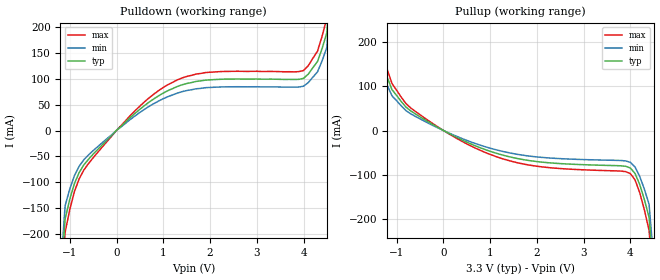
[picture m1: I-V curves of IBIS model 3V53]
[IBIS Ver]   2.1
[File name]   171601_3.ibs
[File Rev]   2.0
[Date]   8/4/03
[Source]   ICS MicroClock Applications Engineering 2
[Disclaimer] This information is for modeling purposes only, and is
(C) Copyright Integrated Circuit Systems, Inc. 1997-2003
   All rights reserved
ICS hereby grants the user of this IBIS model a non-exclusive,
nontransferable license to use this IBIS model under the following terms.
Before using this IBIS model, the user should read this license.
If the user does not accept these terms,  the IBIS model should be
returned to ICS within 30 days.
   The user is granted this license only to use the IBIS model and
is not granted rights to sell, load, rent, lease or license the IBIS
model in whole or in part, or in modified form to anyone other than
user. User may modify the IBIS model to suit its specific
applications but rights to derivative works and such modifications
shall belong to ICS.
   This IBIS model is provided on an "AS IS" basis and ICS makes
absolutely no warranty with respect to the information contained
herein. ICS DISCLAIMS AND CUSTOMER WAIVES ALL WARRANTIES, EXPRESS
OR IMPLIED, INCLUDING WARRANTIES OF MERCHANTABILITY OR FITNESS FOR
A PARTICULAR PURPOSE. The entire risk as to quality and performance
is with the Customer. ACCORDINGLY, IN NO EVENT SHALL THE COMPANY BE
LIABLE FOR ANY DAMAGES, WHETHER IN CONTRACT OR TORT,INCLUDING ANY
LOST PROFITS OR OTHER INCIDENTAL, CONSEQUENTIAL, EXEMPLARY, OR
PUNITIVE DAMAGES ARISING OUT OF THE USE OR APPLICATION OF THE IBIS
model provided in this package. Further, ICS reserves the right to
make changes without notice to any product herein to improve
reliability, function, or design. ICS does not convey any license
under patent rights or any other intellectual property rights,
including those of third parties.
   ICS is not obligated to provide maintenance or support
for the licensed IBIS model.
[Component]   MK1716-01
[Manufacturer] Integrated Circuit Systems Inc.
[Package]
|   typ   min   max
R_pkg   40m   35m   45m
L_pkg   1.65nH   1.35nH   1.95nH
C_pkg   0.24pF   0.14pF   0.34pF
[pin]   signal_name   model_name   R_pin   L_pin   C_pin
   4   REFOUT   3V53
  10   CLKA   3V53
  11   CLKA   3V53
  12   CLKA   3V53
  13   CLKA   3V53
  16   CLKB   3V53
  17   CLKB   3V53
  18   CLKB   3V53
  19   CLKB   3V53
| Models and submodels in the file (1): 3V53 (Output)
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|   MK1716-01 3.3V Clock Drive Model
| This model is suitable for all output pins on the
| MK1716-01
[Model]   3V53
Model_type   Output
Polarity   Non-Inverting
|   typ   min   max
C_comp   5pF   4pF   6pF
|   typ   min   max
[Voltage range]  3.3V   3.15V   3.45V
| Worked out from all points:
|   slope of the pulldown table from 0 to 0.495 V, typ, clamps not added: 12.3 ohm
|   slope of the pullup table from 0 to 0.495 V, typ, clamps not added: 18.9 ohm
[pulldown]
|Voltage   I (typ)   I (min)   I (max)
-3.3V     -3A        -3A        -3A
-1.1V     -170.4mA   -144.9mA   -196mA
-900mV    -102mA     -86.67mA   -117.3mA
-600mV    -55.36mA   -47.06mA   -63.66mA
500mV     41.05mA    34.89mA    47.2mA
1.3V      84.84mA    72.12mA    97.57mA
2V        97.7mA     83.04mA    112.4mA
4V        100.5mA    85.44mA    115.6mA
4.3V      133.1mA    113.2mA    153.1mA
4.4V      158.6mA    134.8mA    182.4mA
4.5V      188.8mA    160.5mA    217.1mA
6.6V      3A         3A         3A
[pullup]
|Voltage I (typ)   I (min)   I (max)
-3.3V     3A         3A         3A
-1.5V     200.2mA    170.1mA    230.2mA
-1.4V     182.5mA    155.1mA    209.8mA
-1.1V     92.5mA     78.62mA    106.4mA
-800mV    52.88mA    44.95mA    60.82mA
400mV     -21.43mA   -18.21mA   -24.64mA
1.7V      -65.72mA   -55.86mA   -75.57mA
4V        -84.83mA   -72.11mA   -97.56mA
4.1V      -97.17mA   -82.59mA   -111.7mA
4.2V      -122.3mA   -103.9mA   -140.6mA
4.4V      -196.5mA   -167mA     -226mA
6.6V      -3A        -3A        -3A
[Ramp]
|   typ   min   max
dV/dt_r   1.36/0.77n   1.29/0.85n   1.43/0.69n
dV/dt_f   1.65/0.51n   1.53/0.56n   1.73/0.46n
